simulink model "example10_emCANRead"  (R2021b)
settings: Solver=FixedStepAuto  StartTime=0  StopTime=inf  FixedStep=0.5  RelTol=1e-3  EnableMultiTasking=on
undefined symbols (not defined in the file or in its folder): based, Big, bool, classic, dsPic33, Endian, Little, MCC, Microchip, PIC24
libraries: embeddedCreatorLib x9, emCANLib x4, emMBSlaveLib x1

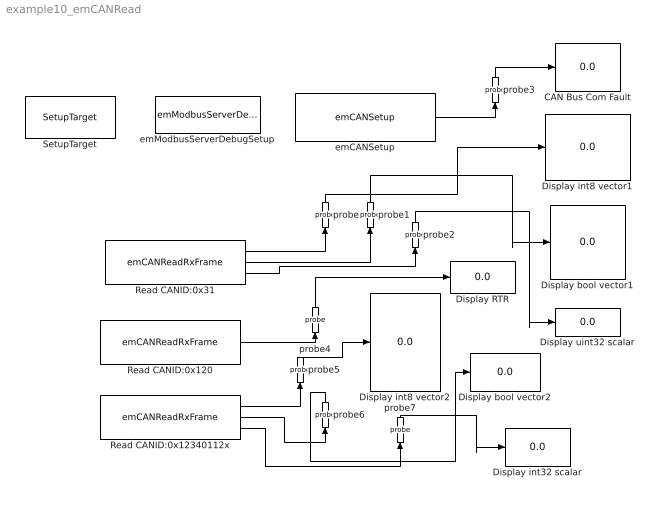
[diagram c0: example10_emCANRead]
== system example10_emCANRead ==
  CAN Bus Com Fault : Display
  Display RTR : Display
  Display bool vector1 : Display
  Display bool vector2 : Display
  Display int32 scalar : Display
  Display int8 vector1 : Display
  Display int8 vector2 : Display
  Display uint32 scalar : Display
  Read CANID:0x120 : emCANLib/emCANReadRxFrame  c_CAN_DeviceNo=1  c_SettingFormat="CAN ID  in Hex Data format"  c_ReceivedType=Standard 11 bits CAN ID short frame  c_CANID=120  c_RTR=on  c_DataType=[int8*3 bool*4 uint32 ]  c_Endian=Little-Endian  c_OutputQty="[3  4  1]"  c_OutputType="[2  8  7]"  c_sampleTime=-1
  Read CANID:0x12340112x : emCANLib/emCANReadRxFrame  c_CAN_DeviceNo=1  c_SettingFormat="CAN ID  in Hex Data format"  c_ReceivedType=Extended 29 bits CAN ID long frame  c_CANID=12340112  c_RTR=off  c_DataType=[int8*5 bool*2 int32*2 ]  c_Endian=Big-Endian  c_OutputQty="[5  2  2]"  c_OutputType="[2  8  6]"  c_sampleTime=-1
  Read CANID:0x31 : emCANLib/emCANReadRxFrame  c_CAN_DeviceNo=1  c_SettingFormat="CAN ID  in Hex Data format"  c_ReceivedType=Standard 11 bits CAN ID short frame  c_CANID=31  c_RTR=off  c_DataType=[int8*3 bool*4 uint32 ]  c_Endian=Little-Endian  c_OutputQty="[3  4  1]"  c_OutputType="[2  8  7]"  c_sampleTime=-1
  SetupTarget : embeddedCreatorLib/SetupTarget  Tag=SetupTarget  Priority=0  c_platform=Microchip PIC24/dsPic33 based on MCC classic  c_debug=on
  emCANSetup : emCANLib/emCANSetup  Tag=emCANBus  c_CAN_DeviceNo=1  c_saved_SettingFormat=1  c_SettingFormat=Settings in Hex Data format  c_Mask0=7F0  c_Mask1=1FFF00FFX  c_Mask2=7F0  c_CANID_short=[120,31,50124X]  c_CANID_long=[12340112X]  c_FrameNoWay=1-based frame No  c_MaxFrameQty=8  c_enableSync=on  c_Sync_RxCANID=12340218X  c_Com_Fault_detection_Time=200  c_ASeq_QTY=31  c_BSeq_QTY=0  c_CSeq_QTY=0  c_RxStdShort_listData=49  c_RxExtShort_listData=327972  c_RxStdLong_listData=-1  c_RxExtLong_listData=305398034  c_RxStdSyncData=-1  c_RxExtSyncData=305398296  c_txChaanelA_DataLength="\"\""  c_txChaanelB_DataLength="\"\""  c_txChaanelC_DataLength="\"\""  c_sampleTime=-1
  emModbusServerDebugSetup : emMBSlaveLib/emModbusServerDebugSetup  Tag=emModbusSlaveSetup  c_objID=0  c_uartNo=2  c_baudrate=19200  c_serverID=1  c_baudrate4PC=19200  c_forceLongerSpace=on  c_holdingRegsQTY=0  c_minHoldingAddr=789  c_inputRegsQTY=0  c_minInputRegAddr=20  c_coilRegsQTY=0  c_minCoilAddr=30  c_discreteRegsQTY=0  c_minDiscreteAddr=40  c_enableDebug=on  c_breakpointMaxQTY=100  c_probeMaxWordQTY=200  c_emWaitQTY=0  g_COMPortNo=COM5  c_Name_method=By physical port name and bit number  c_PortName=B  c_BitNo=11  c_TxEnable485="\"LATBbits.LATB11\""  c_TxEnable485Polarity=on
  probe : embeddedCreatorLib/probe  Tag=emProbe  c_ObjID=4  c_serverID=1  c_UartNo=1  c_StartAddr=17  c_ConstantDataSource=off
  probe1 : embeddedCreatorLib/probe  Tag=emProbe  c_ObjID=3  c_serverID=1  c_UartNo=1  c_StartAddr=13  c_ConstantDataSource=off
  probe2 : embeddedCreatorLib/probe  Tag=emProbe  c_ObjID=5  c_serverID=1  c_UartNo=1  c_StartAddr=20  c_ConstantDataSource=off
  probe3 : embeddedCreatorLib/probe  Tag=emProbe  c_ObjID=7  c_serverID=1  c_UartNo=1  c_StartAddr=23  c_ConstantDataSource=off
  probe4 : embeddedCreatorLib/probe  Tag=emProbe  c_ObjID=6  c_serverID=1  c_UartNo=1  c_StartAddr=22  c_ConstantDataSource=off
  probe5 : embeddedCreatorLib/probe  Tag=emProbe  c_ObjID=0  c_serverID=1  c_UartNo=1  c_StartAddr=2  c_ConstantDataSource=off
  probe6 : embeddedCreatorLib/probe  Tag=emProbe  c_ObjID=1  c_serverID=1  c_UartNo=1  c_StartAddr=7  c_ConstantDataSource=off
  probe7 : embeddedCreatorLib/probe  Tag=emProbe  c_ObjID=2  c_serverID=1  c_UartNo=1  c_StartAddr=9  c_ConstantDataSource=off
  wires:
  probe1/1 -> Display bool vector1/1
  Read CANID:0x31/1 -> probe/1
  probe/1 -> Display int8 vector1/1
  Read CANID:0x31/2 -> probe1/1
  Read CANID:0x31/3 -> probe2/1
  probe2/1 -> Display uint32 scalar/1
  emCANSetup/1 -> probe3/1
  probe3/1 -> CAN Bus Com Fault/1
  Read CANID:0x120/1 -> probe4/1
  probe4/1 -> Display RTR/1
  Read CANID:0x12340112x/1 -> probe5/1
  probe5/1 -> Display int8 vector2/1
  Read CANID:0x12340112x/2 -> probe6/1
  probe6/1 -> Display bool vector2/1
  Read CANID:0x12340112x/3 -> probe7/1
  probe7/1 -> Display int32 scalar/1
